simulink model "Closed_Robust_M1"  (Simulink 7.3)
settings: Solver=ode45  StartTime=0.0  StopTime=200  RelTol=1e-3
undefined symbols (not defined in the file or in its folder): Acl, Bcl, Ccl, Dcl

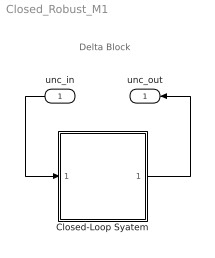
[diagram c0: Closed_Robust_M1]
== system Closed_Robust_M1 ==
  note: Delta Block
  unc_in : Inport
  Closed-Loop Syatem : Subsystem
  unc_out : Outport
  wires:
  Closed-Loop Syatem/1(unc_out) -> unc_out/1
  unc_in/1 -> Closed-Loop Syatem/1(unc_in)

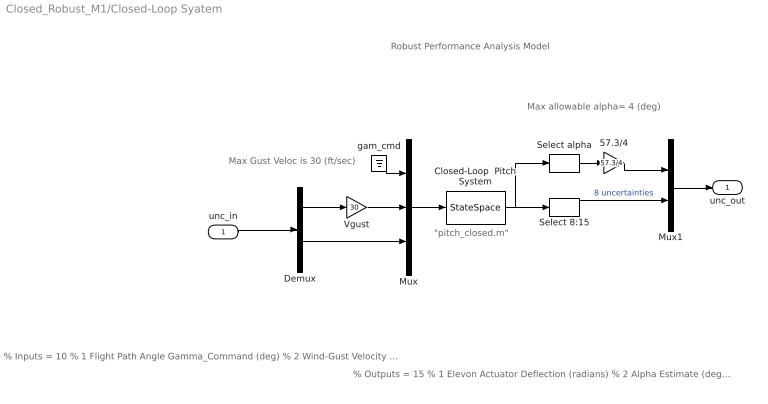
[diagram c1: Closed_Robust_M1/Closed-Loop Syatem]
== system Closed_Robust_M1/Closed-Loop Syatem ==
  note: % Outputs = 15 % 1 Elevon Actuator Deflection (radians) % 2 Alpha Estimate (deg) % 3 Pitch Attitude (thet-123) (radians) % 4 Pitch Rate (q-body) (rad/sec) % 5 Angle of attack, alfa, (radians) % 6 Accelerom # 2, (along Z), (ft/sec^2) % 7 Alpha Sensed at Vane # 1 (radian) % 8 Cm_alpha : -36.364 % Variation % 9 Cz_alpha : -21.875 % Variation % 10 Cm_0 : -27.027 % Variation % 11 CZ_0 : -50.000 % Variation % 12 I_yy : 4.232 % Variation % 13 Xcg locat: 1.909 % Variation % 14 Cz_surf 1: -32.184 % Variation % 15 Cm_surf 1: -34.722 % Variation
  note: % Inputs = 10 % 1 Flight Path Angle Gamma_Command (deg) % 2 Wind-Gust Velocity pre-shaped (ft/sec) % 3 Cm_alpha : -36.364 % Variation % 4 Cz_alpha : -21.875 % Variation % 5 Cm_0 : -27.027 % Variation % 6 CZ_0 : -50.000 % Variation % 7 I_yy : 4.232 % Variation % 8 Xcg locat: 1.909 % Variation % 9 Cz_surf 1: -32.184 % Variation % 10 Cm_surf 1: -34.722 % Variation
  note: Robust Performance Analysis Model
  note: Max allowable alpha= 4 (deg)
  note: Max Gust Veloc is 30 (ft/sec)
  note: "pitch_closed.m"
  unc_in : Inport
  57.3/4 : Gain  Gain=57.3/4  ParameterDataType=fixdt(1, 16)  ParameterScaling=2^0  OutDataType=fixdt(1, 16)  OutScaling=2^0
  Closed-Loop  Pitch System : StateSpace  A=Acl  B=Bcl  C=Ccl  D=Dcl
  Demux : Demux  Outputs=[1,8]
  Mux : Mux  Inputs=[1, 1, 8]
  Mux1 : Mux  Inputs="[1,  8]"
  Select 8:15 : Selector  InputPortWidth=15  IndexOptions=Index vector (dialog)  Indices=[8:15]  OutputSizes=1
  Select alpha : Selector  InputPortWidth=15  IndexOptions=Index vector (dialog)  Indices=[5]  OutputSizes=1
  Vgust : Gain  Gain=30  ParameterDataType=fixdt(1, 16)  ParameterScaling=2^0  OutDataType=fixdt(1, 16)  OutScaling=2^0
  gam_cmd : Ground
  unc_out : Outport
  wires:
  Closed-Loop  Pitch System/1 -> Select 8:15/1, Select alpha/1
  Mux/1 -> Closed-Loop  Pitch System/1
  gam_cmd/1 -> Mux/1
  Demux/2 -> Mux/3
  Demux/1 -> Vgust/1
  unc_in/1 -> Demux/1
  Select 8:15/1 -> Mux1/2  "8 uncertainties"
  Select alpha/1 -> 57.3/4/1
  Mux1/1 -> unc_out/1
  Vgust/1 -> Mux/2
  57.3/4/1 -> Mux1/1
